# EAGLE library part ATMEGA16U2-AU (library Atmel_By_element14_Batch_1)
8-bit Microcontroller
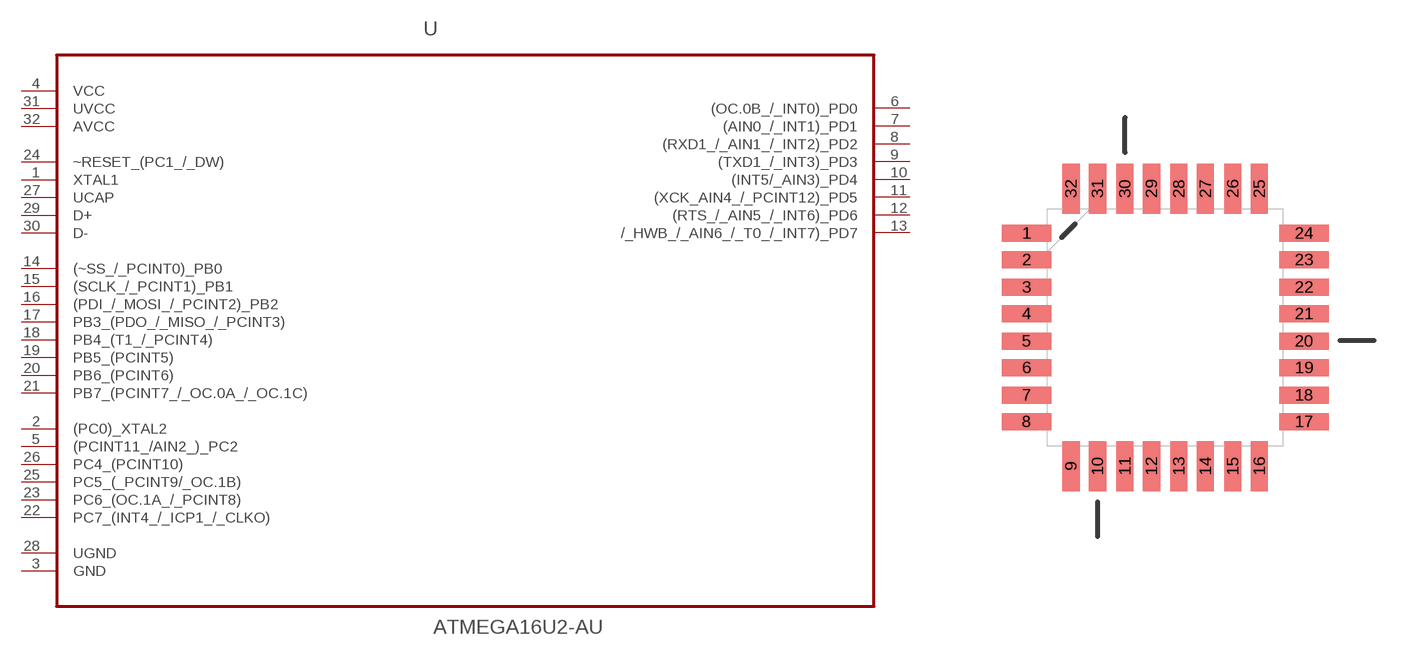
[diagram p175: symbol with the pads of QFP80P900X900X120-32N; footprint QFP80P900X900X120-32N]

Designator prefix U

## ATMEGA16U2-AU (MPN: ATMEGA16U2-AU; OC_FARNELL: 1841607; OC_NEWARK: 12T1292; PACKAGE: QFP-32; SUPPLIER: Atmel)  [QFP80P900X900X120-32N]
1  XTAL1  in
2  (PC0)_XTAL2  out
3  GND  pas
4  VCC  pwr
5  (PCINT11_/AIN2_)_PC2
6  (OC.0B_/_INT0)_PD0
7  (AIN0_/_INT1)_PD1
8  (RXD1_/_AIN1_/_INT2)_PD2
9  (TXD1_/_INT3)_PD3
10  (INT5/_AIN3)_PD4
11  (XCK_AIN4_/_PCINT12)_PD5
12  (RTS_/_AIN5_/_INT6)_PD6
13  /_HWB_/_AIN6_/_T0_/_INT7)_PD7
14  (~SS_/_PCINT0)_PB0
15  (SCLK_/_PCINT1)_PB1
16  (PDI_/_MOSI_/_PCINT2)_PB2
17  PB3_(PDO_/_MISO_/_PCINT3)
18  PB4_(T1_/_PCINT4)
19  PB5_(PCINT5)
20  PB6_(PCINT6)
21  PB7_(PCINT7_/_OC.0A_/_OC.1C)
22  PC7_(INT4_/_ICP1_/_CLKO)
23  PC6_(OC.1A_/_PCINT8)
24  ~RESET_(PC1_/_DW)  in
25  PC5_(_PCINT9/_OC.1B)
26  PC4_(PCINT10)
27  UCAP  pas
28  UGND  pas
29  D+  pas
30  D-  pas
31  UVCC  pwr
32  AVCC  pwr

## Footprint QFP80P900X900X120-32N (pad centres in mm)
smd 1.473 x 0.508: 1 -4.115,2.794; 2 -4.115,2.007; 3 -4.115,1.194; 4 -4.115,0.406; 5 -4.115,-0.406; 6 -4.115,-1.194; 7 -4.115,-2.007; 8 -4.115,-2.794; 17 4.115,-2.794; 18 4.115,-2.007; 19 4.115,-1.194; 20 4.115,-0.406; 21 4.115,0.406; 22 4.115,1.194; 23 4.115,2.007; 24 4.115,2.794
smd 0.508 x 1.473: 9 -2.794,-4.115; 10 -2.007,-4.115; 11 -1.194,-4.115; 12 -0.406,-4.115; 13 0.406,-4.115; 14 1.194,-4.115; 15 2.007,-4.115; 16 2.794,-4.115; 25 2.794,4.115; 26 2.007,4.115; 27 1.194,4.115; 28 0.406,4.115; 29 -0.406,4.115; 30 -1.194,4.115; 31 -2.007,4.115; 32 -2.794,4.115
